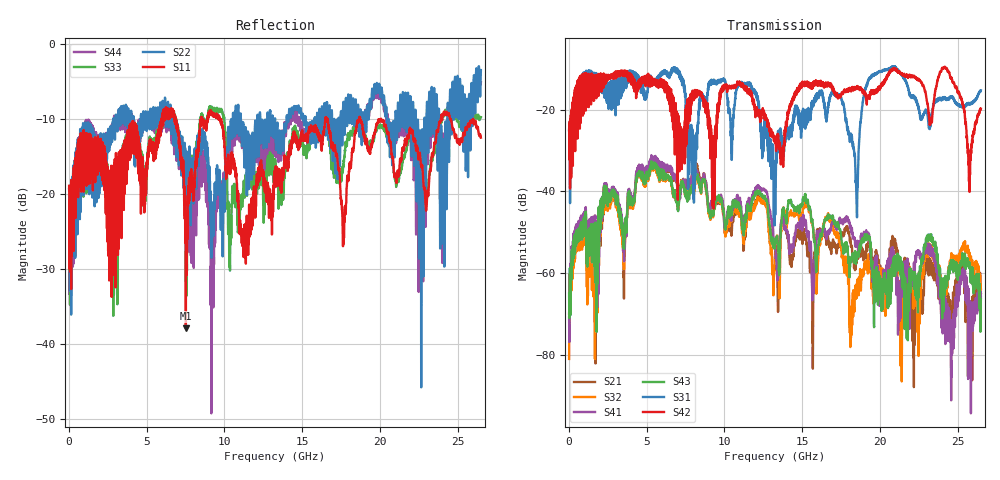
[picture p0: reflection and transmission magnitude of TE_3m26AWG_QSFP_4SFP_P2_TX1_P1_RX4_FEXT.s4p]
!Agilent Technologies,N5222A,MY51421691,A.10.00.00
!Agilent N5222A: A.10.00.00
!Date: Friday, January 30, 2015 12:37:08
!Correction: S11(Full 4 Port(1,2,3,4))
!S12(Full 4 Port(1,2,3,4))
!S13(Full 4 Port(1,2,3,4))
!S14(Full 4 Port(1,2,3,4))
!S21(Full 4 Port(1,2,3,4))
!S22(Full 4 Port(1,2,3,4))
!S23(Full 4 Port(1,2,3,4))
!S24(Full 4 Port(1,2,3,4))
!S31(Full 4 Port(1,2,3,4))
!S32(Full 4 Port(1,2,3,4))
!S33(Full 4 Port(1,2,3,4))
!S34(Full 4 Port(1,2,3,4))
!S41(Full 4 Port(1,2,3,4))
!S42(Full 4 Port(1,2,3,4))
!S43(Full 4 Port(1,2,3,4))
!S44(Full 4 Port(1,2,3,4))
!S4P File: Measurements: <S11,S12,S13,S14>,
!<S21,S22,S23,S24>,
!<S31,S32,S33,S34>,
!<S41,S42,S43,S44>:
# Hz S  dB  R 50.0
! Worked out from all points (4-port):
!   2650 points, 10 MHz to 26.5 GHz, reference 50 ohm
!   strongest paths, dB at 10 MHz, 6.63 GHz, 13.26 GHz, 19.88 GHz, 26.5 GHz:
!     S42: -25.0, -19.3, -26.9, -15.1, -19.7
!     S31: -25.0, -10.3, -36.3, -10.7, -15.2
!     S43: -65.0, -38.4, -53.0, -67.8, -66.5
!     S41: -70.9, -34.4, -53.2, -61.8, -65.7
!     S32: -81.1, -38.8, -55.1, -62.4, -65.2
!     S21: -70.0, -35.0, -51.7, -59.0, -63.9
!   lowest |S11| = -38.0 dB at 7.52 GHz (marker M1), VSWR 1.03, Z = 51.2 + j0.31 ohm
!   |S11| at or under -10 dB: start of sweep to 5.956 GHz; 9.72 GHz to 16.5 GHz (6.775 GHz wide, 51.7 % of centre); 18.73 GHz to 23.92 GHz (5.187 GHz wide, 24.3 % of centre)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
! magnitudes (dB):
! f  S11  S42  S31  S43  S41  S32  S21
! 10 MHz  -18.9  -25.0  -25.0  -65.0  -70.9  -81.1  -70.0
! 2.31 GHz  -14.1  -11.5  -12.6  -43.0  -42.6  -44.6  -44.5
! 7.52 GHz  -38.0  -24.1  -19.8  -39.6  -37.0  -39.4  -37.4
! 17.33 GHz  -16.8  -17.1  -16.4  -48.2  -48.3  -50.5  -53.6
! 18.49 GHz  -11.1  -14.8  -41.8  -57.0  -53.6  -64.5  -57.3
! 19.59 GHz  -12.3  -15.1  -11.4  -62.6  -59.8  -61.4  -56.9
! 26.5 GHz  -12.5  -19.7  -15.2  -66.5  -65.7  -65.2  -63.9
